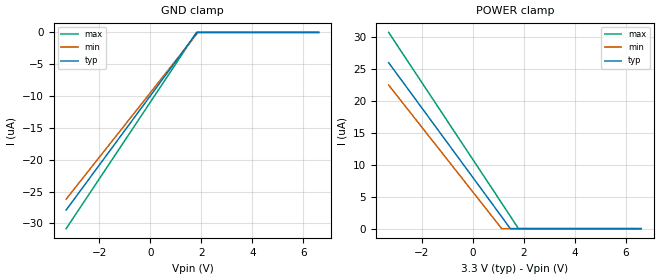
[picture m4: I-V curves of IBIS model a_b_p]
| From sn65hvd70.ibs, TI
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|   a_b Model
[Model]   a_b_p
Model_type   Input
Vinl = 0.8
Vinh = 2
|   typ   min   max
|   (nom PVT)   (fast PVT)   (slow PVT)
|Average
C_comp   3.733e-12   3.726e-12   3.785e-12
| Where nom  PVT is Nominal Process, 3.3V, 27C
|   Fast PVT is Strong Process,  3.6V, -40C
|   Slow PVT is Weak Process,   3V, 150C
[Voltage Range]   3.3   3   3.6
|Ambient Temperature   25   125   -40
|Junction Temperature
[Temperature Range]   27   150   -40
[Power Clamp Reference]   3.3   3   3.6
[GND Clamp Reference]   0   0   0
[GND Clamp]
|   Voltage   I(typ)   I(min)   I(max)
-3.3V     -27.91uA   -26.2uA    -30.84uA
1.808V    -113nA     -299.4nA   -15.76nA
1.866V    0A         0A         0A
6.6V      0A         0A         0A
[POWER Clamp]
|   Voltage   I(typ)   I(min)   I(max)
-3.3V     25.96uA    22.46uA    30.7uA
1.131V    1.86uA     0A         4.006uA
1.468V    13.45nA    0A         1.955uA
1.787V    0A         0A         13.55nA
6.6V      0A         0A         0A
